| TEXAS INSTRUMENTS INCORPORATED
| Standard Linear and Logic Group
| IBIS Model of SN74ALVCH16973
| 8-BIT BUS TRANSCEIVER AND TRANSPARENT D-TYPE LATCH WITH FOUR
| INDEPENDENT BUFFERS
| This file contains package information for the following:
|  SSOP 48-pin (DL) package as [Component] ALVCH16973_DL
|  TSSOP 48-pin (DGG) package as [Component] ALVCH16973_DGG
|  TVSOP 48-pin (DGV) package as [Component] ALVCH16973_DGV
| This device can be powered at the following Vccs:
|  1.8 volt Vcc
|  2.5 volt Vcc
|  3.3 volt Vcc
| This file provides unique models under the [Model Selector] for each Vcc.
| For operation at a specific Vcc, select the appropriate model after each
| [Model Selector] keyword.
[IBIS Ver]   3.2
[Comment char]  |_char
[File Name]   sn74alvch16973.ibs
[File Rev]   1.1 | x_die
[Date]   March 1, 2003
[Source]   Data created from TI-SPICE simulations at TI-SLL.
[Notes]   The following is an IBIS list for the ALVCH16973.
   Please contact sllibis@ti.com with questions and
   comments concerning SLL IBIS models.
   - Due to presence of bus hold at input, GND-clamp curves
   have non-monotonic warnings.
   - Power-clamp data has been deleted from the control pin
   models since there is no power-clamp diode.
[Disclaimer] Property of Texas Instruments Incorporated.  Unauthorized
   reproduction and/or distribution is strictly prohibited.
   This product is protected under copyright law.
   Created  2002, (C) Copyright  2002, Texas Instruments
   Incorporated, All Rights Reserved
   UNLESS THERE IS A SIGNED, WRITTEN AGREEMENT TO THE
   CONTRARY, TEXAS INSTRUMENTS (TI) IS PROVIDING THE IBIS
   MODELS  AND WITHOUT ANY WARRANTY, EXPRESSED OR
   IMPLIED.  TI assumes no liability for:
   1) the accuracy of the IBIS models provided to your
   company;
   2) the proper functioning of these IBIS Models in your
   design or for any resulting applications; or
   3) infringement of patents, copyrights or intellectual
   property rights resulting from your use of these IBIS
   models.
   TI provides IBIS Models as a service to our customers.
   You and your company shall not distribute, sell or give
   these models to anyone else without prior written
   permission from TI.
   TI reserves the right to make changes to our products or
   to discontinue any semiconductor product or service
   without notice, and advises our customers to obtain the
   latest version of relevant information to verify, before
   placing orders, that the information being relied on is
   current.
   Please be aware that your receipt and use of the IBIS
   information provided shall serve as acceptance of these
   terms and conditions.  If you do not accept these terms,
   you should return or destroy the IBIS models and any
   other accompanying information immediately.
| Component ALVCH16973_DL 48-pin SSOP
[Component]   ALVCH16973_DL
[Manufacturer]   Texas Instruments, Inc.
[Package]
|   typ   min   max
R_pkg   4.800e-02   3.800e-02   5.300e-02
L_pkg   6.046e-09   5.084e-09   7.968e-09
C_pkg   8.130e-13   5.690e-13   1.157e-12
[Pin]   signal_name   model_name   R_pin   L_pin   C_pin
1   NTOE   ALVCH16973_NTOE   4.600e-02   7.968e-09   1.017e-12
2   D1   ALVCH16973_D   4.400e-02   7.299e-09   1.157e-12
3   A1   ALVCH16973_AIO   4.300e-02   6.765e-09   1.058e-12
4   GND   GND   4.100e-02   6.269e-09   9.330e-13
5   Y1   ALVCH16973_YOUT   3.800e-02   5.856e-09   8.290e-13
6   A2   ALVCH16973_AIO   4.600e-02   5.802e-09   7.900e-13
7   VCC   POWER   5.000e-02   5.656e-09   7.380e-13
8   D2   ALVCH16973_D   5.300e-02   5.500e-09   6.430e-13
9   A3   ALVCH16973_AIO   5.200e-02   5.304e-09   6.060e-13
10   GND   GND   5.300e-02   5.189e-09   5.830e-13
11   Y2   ALVCH16973_YOUT   5.100e-02   5.084e-09   5.690e-13
12   A4   ALVCH16973_AIO   5.300e-02   5.862e-09   8.330e-13
13   D3   ALVCH16973_D   5.300e-02   5.862e-09   8.330e-13
14   A5   ALVCH16973_AIO   5.100e-02   5.084e-09   5.690e-13
15   GND   GND   5.300e-02   5.189e-09   5.830e-13
16   Y3   ALVCH16973_YOUT   5.200e-02   5.304e-09   6.060e-13
17   A6   ALVCH16973_AIO   5.300e-02   5.500e-09   6.430e-13
18   VCC   POWER   5.000e-02   5.656e-09   7.380e-13
19   D4   ALVCH16973_D   4.600e-02   5.802e-09   7.900e-13
20   A7   ALVCH16973_AIO   3.800e-02   5.856e-09   8.290e-13
21   GND   GND   4.100e-02   6.269e-09   9.330e-13
22   A8   ALVCH16973_AIO   4.300e-02   6.765e-09   1.058e-12
23   Y4   ALVCH16973_YOUT   4.400e-02   7.299e-09   1.157e-12
24   LE   ALVCH16973_LE   4.600e-02   7.968e-09   1.017e-12
25   NLOE   ALVCH16973_NLOE   4.600e-02   7.968e-09   1.017e-12
26   B8   ALVCH16973_BIO   4.400e-02   7.299e-09   1.157e-12
27   Q8   ALVCH16973_QOUT   4.300e-02   6.765e-09   1.058e-12
28   GND   GND   4.100e-02   6.269e-09   9.330e-13
29   Q7   ALVCH16973_QOUT   3.800e-02   5.856e-09   8.290e-13
30   B7   ALVCH16973_BIO   4.600e-02   5.802e-09   7.900e-13
31   VCC   POWER   5.000e-02   5.656e-09   7.380e-13
32   Q6   ALVCH16973_QOUT   5.300e-02   5.500e-09   6.430e-13
33   B6   ALVCH16973_BIO   5.200e-02   5.304e-09   6.060e-13
34   GND   GND   5.300e-02   5.189e-09   5.830e-13
35   Q5   ALVCH16973_QOUT   5.100e-02   5.084e-09   5.690e-13
36   B5   ALVCH16973_BIO   5.300e-02   5.862e-09   8.330e-13
37   Q4   ALVCH16973_QOUT   5.300e-02   5.862e-09   8.330e-13
38   B4   ALVCH16973_BIO   5.100e-02   5.084e-09   5.690e-13
39   GND   GND   5.300e-02   5.189e-09   5.830e-13
40   Q3   ALVCH16973_QOUT   5.200e-02   5.304e-09   6.060e-13
41   B3   ALVCH16973_BIO   5.300e-02   5.500e-09   6.430e-13
42   VCC   POWER   5.000e-02   5.656e-09   7.380e-13
43   Q2   ALVCH16973_QOUT   4.600e-02   5.802e-09   7.900e-13
44   B2   ALVCH16973_BIO   3.800e-02   5.856e-09   8.290e-13
45   GND   GND   4.100e-02   6.269e-09   9.330e-13
46   Q1   ALVCH16973_QOUT   4.300e-02   6.765e-09   1.058e-12
47   B1   ALVCH16973_BIO   4.400e-02   7.299e-09   1.157e-12
48   DIR   ALVCH16973_DIR   4.600e-02   7.967e-09   1.017e-12
| Component ALVCH16973_DGG 48-pin TSSOP
[Component]   ALVCH16973_DGG
[Manufacturer]   Texas Instruments, Inc.
[Package]
|   typ   min   max
R_pkg   6.200e-02   5.000e-02   7.800e-02
L_pkg   3.527e-09   3.128e-09   4.255e-09
C_pkg   5.300e-13   4.170e-13   6.850e-13
[Pin]   signal_name   model_name   R_pin   L_pin   C_pin
1   NTOE   ALVCH16973_NTOE   5.000e-02   4.250e-09   6.710e-13
2   D1   ALVCH16973_D   5.700e-02   3.956e-09   6.740e-13
3   A1   ALVCH16973_AIO   7.100e-02   3.922e-09   6.190e-13
4   GND   GND   7.800e-02   3.841e-09   6.180e-13
5   Y1   ALVCH16973_YOUT   5.600e-02   3.535e-09   5.550e-13
6   A2   ALVCH16973_AIO   5.800e-02   3.464e-09   5.030e-13
7   VCC   POWER   6.000e-02   3.362e-09   4.980e-13
8   D2   ALVCH16973_D   6.100e-02   3.293e-09   4.620e-13
9   A3   ALVCH16973_AIO   6.300e-02   3.240e-09   4.550e-13
10   GND   GND   6.300e-02   3.175e-09   4.420e-13
11   Y2   ALVCH16973_YOUT   6.400e-02   3.153e-09   4.290e-13
12   A4   ALVCH16973_AIO   6.500e-02   3.128e-09   4.180e-13
13   D3   ALVCH16973_D   6.500e-02   3.128e-09   4.180e-13
14   A5   ALVCH16973_AIO   6.400e-02   3.154e-09   4.290e-13
15   GND   GND   6.300e-02   3.174e-09   4.420e-13
16   Y3   ALVCH16973_YOUT   6.300e-02   3.241e-09   4.550e-13
17   A6   ALVCH16973_AIO   6.100e-02   3.293e-09   4.620e-13
18   VCC   POWER   6.000e-02   3.362e-09   4.970e-13
19   D4   ALVCH16973_D   5.800e-02   3.464e-09   5.030e-13
20   A7   ALVCH16973_AIO   5.600e-02   3.537e-09   5.600e-13
21   GND   GND   7.700e-02   3.839e-09   6.260e-13
22   A8   ALVCH16973_AIO   7.100e-02   3.917e-09   6.270e-13
23   Y4   ALVCH16973_YOUT   5.800e-02   3.955e-09   6.850e-13
24   LE   ALVCH16973_LE   5.200e-02   4.255e-09   6.790e-13
25   NLOE   ALVCH16973_NLOE   5.100e-02   4.254e-09   6.760e-13
26   B8   ALVCH16973_BIO   5.800e-02   3.957e-09   6.790e-13
27   Q8   ALVCH16973_QOUT   7.100e-02   3.920e-09   6.210e-13
28   GND   GND   7.800e-02   3.843e-09   6.220e-13
29   Q7   ALVCH16973_QOUT   5.600e-02   3.539e-09   5.600e-13
30   B7   ALVCH16973_BIO   5.800e-02   3.466e-09   5.030e-13
31   VCC   POWER   6.000e-02   3.363e-09   4.970e-13
32   Q6   ALVCH16973_QOUT   6.100e-02   3.294e-09   4.620e-13
33   B6   ALVCH16973_BIO   6.300e-02   3.241e-09   4.540e-13
34   GND   GND   6.300e-02   3.175e-09   4.410e-13
35   Q5   ALVCH16973_QOUT   6.400e-02   3.153e-09   4.290e-13
36   B5   ALVCH16973_BIO   6.500e-02   3.129e-09   4.170e-13
37   Q4   ALVCH16973_QOUT   6.500e-02   3.129e-09   4.170e-13
38   B4   ALVCH16973_BIO   6.400e-02   3.152e-09   4.290e-13
39   GND   GND   6.400e-02   3.176e-09   4.410e-13
40   Q3   ALVCH16973_QOUT   6.300e-02   3.241e-09   4.540e-13
41   B3   ALVCH16973_BIO   6.100e-02   3.293e-09   4.620e-13
42   VCC   POWER   6.000e-02   3.363e-09   4.970e-13
43   Q2   ALVCH16973_QOUT   5.800e-02   3.464e-09   5.030e-13
44   B2   ALVCH16973_BIO   5.600e-02   3.534e-09   5.610e-13
45   GND   GND   7.800e-02   3.841e-09   6.260e-13
46   Q1   ALVCH16973_QOUT   7.100e-02   3.920e-09   6.220e-13
47   B1   ALVCH16973_BIO   5.700e-02   3.955e-09   6.770e-13
48   DIR   ALVCH16973_DIR   5.100e-02   4.252e-09   6.720e-13
| Component ALVCH16973_DGV 48-pin TVSOP
[Component]   ALVCH16973_DGV
[Manufacturer]   Texas Instruments, Inc.
[Package]
|   typ   min   max
R_pkg   7.000e-02   4.900e-02   8.500e-02
L_pkg   3.013e-09   2.743e-09   3.408e-09
C_pkg   3.710e-13   2.940e-13   5.110e-13
[Pin]   signal_name   model_name   R_pin   L_pin   C_pin
1   NTOE   ALVCH16973_NTOE   4.900e-02   3.393e-09   4.970e-13
2   D1   ALVCH16973_D   6.000e-02   3.250e-09   5.020e-13
3   A1   ALVCH16973_AIO   7.700e-02   3.310e-09   4.510e-13
4   GND   GND   8.500e-02   3.299e-09   4.040e-13
5   Y1   ALVCH16973_YOUT   8.300e-02   3.136e-09   3.600e-13
6   A2   ALVCH16973_AIO   7.700e-02   3.019e-09   3.630e-13
7   VCC   POWER   6.500e-02   2.882e-09   3.490e-13
8   D2   ALVCH16973_D   6.600e-02   2.829e-09   3.140e-13
9   A3   ALVCH16973_AIO   6.700e-02   2.796e-09   3.140e-13
10   GND   GND   6.900e-02   2.754e-09   3.080e-13
11   Y2   ALVCH16973_YOUT   7.000e-02   2.753e-09   3.010e-13
12   A4   ALVCH16973_AIO   7.100e-02   2.745e-09   2.940e-13
13   D3   ALVCH16973_D   7.000e-02   2.744e-09   2.940e-13
14   A5   ALVCH16973_AIO   7.000e-02   2.754e-09   3.010e-13
15   GND   GND   6.900e-02   2.754e-09   3.080e-13
16   Y3   ALVCH16973_YOUT   6.700e-02   2.796e-09   3.140e-13
17   A6   ALVCH16973_AIO   6.600e-02   2.829e-09   3.140e-13
18   VCC   POWER   6.500e-02   2.883e-09   3.500e-13
19   D4   ALVCH16973_D   7.500e-02   3.014e-09   3.630e-13
20   A7   ALVCH16973_AIO   8.000e-02   3.128e-09   3.580e-13
21   GND   GND   8.400e-02   3.295e-09   4.030e-13
22   A8   ALVCH16973_AIO   7.800e-02   3.311e-09   4.520e-13
23   Y4   ALVCH16973_YOUT   6.200e-02   3.259e-09   5.010e-13
24   LE   ALVCH16973_LE   5.200e-02   3.404e-09   4.960e-13
25   NLOE   ALVCH16973_NLOE   5.300e-02   3.397e-09   5.050e-13
26   B8   ALVCH16973_BIO   6.200e-02   3.249e-09   5.110e-13
27   Q8   ALVCH16973_QOUT   7.700e-02   3.308e-09   4.530e-13
28   GND   GND   8.200e-02   3.289e-09   4.030e-13
29   Q7   ALVCH16973_QOUT   7.800e-02   3.121e-09   3.590e-13
30   B7   ALVCH16973_BIO   7.400e-02   3.010e-09   3.630e-13
31   VCC   POWER   6.500e-02   2.883e-09   3.490e-13
32   Q6   ALVCH16973_QOUT   6.700e-02   2.829e-09   3.140e-13
33   B6   ALVCH16973_BIO   6.700e-02   2.795e-09   3.140e-13
34   GND   GND   6.900e-02   2.753e-09   3.070e-13
35   Q5   ALVCH16973_QOUT   7.000e-02   2.753e-09   3.010e-13
36   B5   ALVCH16973_BIO   7.000e-02   2.743e-09   2.940e-13
37   Q4   ALVCH16973_QOUT   7.000e-02   2.743e-09   2.940e-13
38   B4   ALVCH16973_BIO   7.000e-02   2.753e-09   3.010e-13
39   GND   GND   6.900e-02   2.754e-09   3.070e-13
40   Q3   ALVCH16973_QOUT   6.800e-02   2.797e-09   3.140e-13
41   B3   ALVCH16973_BIO   6.700e-02   2.830e-09   3.140e-13
42   VCC   POWER   6.400e-02   2.880e-09   3.490e-13
43   Q2   ALVCH16973_QOUT   7.200e-02   3.004e-09   3.620e-13
44   B2   ALVCH16973_BIO   7.800e-02   3.121e-09   3.590e-13
45   GND   GND   8.400e-02   3.296e-09   4.030e-13
46   Q1   ALVCH16973_QOUT   7.700e-02   3.308e-09   4.510e-13
47   B1   ALVCH16973_BIO   6.200e-02   3.258e-09   4.990e-13
48   DIR   ALVCH16973_DIR   5.300e-02   3.408e-09   4.940e-13
| Model ALVCH16973_LE
[Model Selector]   ALVCH16973_LE
ALVCH16973_LE_18   1.8 volt Vcc
ALVCH16973_LE_25   2.5 volt Vcc
ALVCH16973_LE_33   3.3 volt Vcc
| Model ALVCH16973_NLOE
[Model Selector]   ALVCH16973_NLOE
ALVCH16973_NLOE_18   1.8 volt Vcc
ALVCH16973_NLOE_25   2.5 volt Vcc
ALVCH16973_NLOE_33   3.3 volt Vcc
| Model ALVCH16973_DIR
[Model Selector]   ALVCH16973_DIR
ALVCH16973_DIR_18   1.8 volt Vcc
ALVCH16973_DIR_25   2.5 volt Vcc
ALVCH16973_DIR_33   3.3 volt Vcc
| Model ALVCH16973_NTOE
[Model Selector]   ALVCH16973_NTOE
ALVCH16973_NTOE_18   1.8 volt Vcc
ALVCH16973_NTOE_25   2.5 volt Vcc
ALVCH16973_NTOE_33   3.3 volt Vcc
| Model ALVCH16973_D
[Model Selector]   ALVCH16973_D
ALVCH16973_D_18   1.8 volt Vcc
ALVCH16973_D_25   2.5 volt Vcc
ALVCH16973_D_33   3.3 volt Vcc
| Model ALVCH16973_AIO
[Model Selector]   ALVCH16973_AIO
ALVCH16973_AIO_18   1.8 volt Vcc
ALVCH16973_AIO_25   2.5 volt Vcc
ALVCH16973_AIO_33   3.3 volt Vcc
| Model ALVCH16973_BIO
[Model Selector]   ALVCH16973_BIO
ALVCH16973_BIO_18   1.8 volt Vcc
ALVCH16973_BIO_25   2.5 volt Vcc
ALVCH16973_BIO_33   3.3 volt Vcc
| Model ALVCH16973_YOUT
[Model Selector]   ALVCH16973_YOUT
ALVCH16973_YOUT_18   1.8 volt Vcc
ALVCH16973_YOUT_25   2.5 volt Vcc
ALVCH16973_YOUT_33   3.3 volt Vcc
| Model ALVCH16973_QOUT
[Model Selector]   ALVCH16973_QOUT
ALVCH16973_QOUT_18   1.8 volt Vcc
ALVCH16973_QOUT_25   2.5 volt Vcc
ALVCH16973_QOUT_33   3.3 volt Vcc
| Models and submodels in the file (27): ALVCH16973_LE_18 (Input), ALVCH16973_LE_25 (Input), ALVCH16973_LE_33 (Input), ALVCH16973_NLOE_18 (Input), ALVCH16973_NLOE_25 (Input), ALVCH16973_NLOE_33 (Input), ALVCH16973_DIR_18 (Input), ALVCH16973_DIR_25 (Input), ALVCH16973_DIR_33 (Input), ALVCH16973_NTOE_18 (Input), ALVCH16973_NTOE_25 (Input), ALVCH16973_NTOE_33 (Input), ALVCH16973_D_18 (Input), ALVCH16973_D_25 (Input), ALVCH16973_D_33 (Input), ALVCH16973_AIO_18 (I/O), ALVCH16973_AIO_25 (I/O), ALVCH16973_AIO_33 (I/O), ALVCH16973_BIO_18 (I/O), ALVCH16973_BIO_25 (I/O), ALVCH16973_BIO_33 (I/O), ALVCH16973_YOUT_18 (Output), ALVCH16973_YOUT_25 (Output), ALVCH16973_YOUT_33 (Output), ALVCH16973_QOUT_18 (3-state), ALVCH16973_QOUT_25 (3-state), ALVCH16973_QOUT_33 (3-state)
